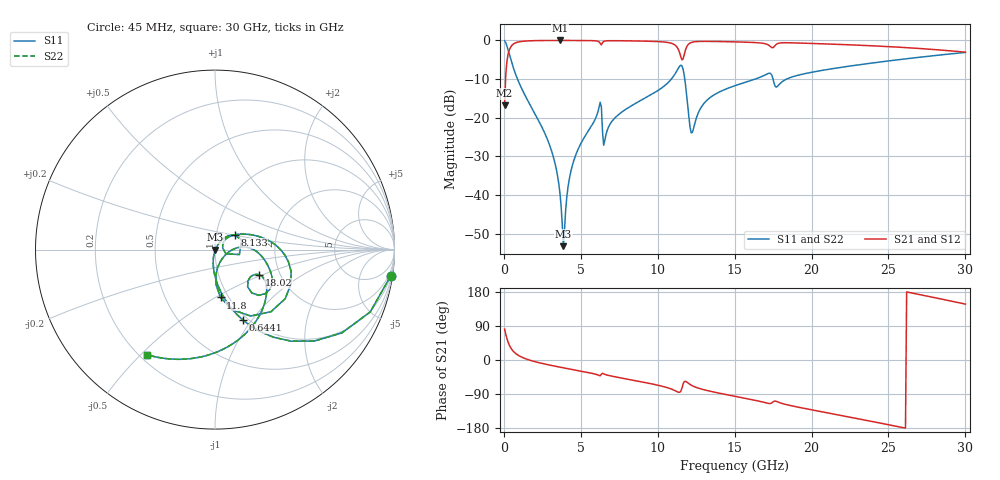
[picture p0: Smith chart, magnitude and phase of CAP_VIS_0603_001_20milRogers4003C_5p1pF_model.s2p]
! S-parameter model data by Modelithics Inc.  support@modelithics.com  813-866-6335  Tampa FL USA
! S-Parameter data specifications:
! Substrate: 20-mil Rogers 4003C, substrate thickness, H=0.508mm, Dielectric constant, Er=3.75
! PCB Mounting Pad Footprint: Pad width, PadW=0.90mm , Pad length, PadL=1.00mm , Pad gap, PadG (edge-to-edge)=1.00mm , Reference planes=3.0mm apart
! Created Wed Nov 18 13:23:11 2015
# hz S ma R 50
! 2 Port Network Data from SP1.SP block
! freq  magS11  angS11  magS21  angS21  magS12  angS12  magS22  angS22
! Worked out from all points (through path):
!   401 points, 45 MHz to 30 GHz, reference 50 ohm
!   highest |S21| = -0.02 dB at 3.64 GHz (marker M1); lowest = -16.8 dB at 45 MHz (marker M2)
!   group delay of S21, straight-line fit = 20.5 ps
!   lowest |S11| = -53.2 dB at 3.864 GHz (marker M3), VSWR 1.00, Z = 50.2 - j0.117 ohm
!   |S11| at or under -10 dB: 881.8 MHz to 10.89 GHz (10 GHz wide, 170 % of centre); 11.75 GHz to 16.34 GHz (4.588 GHz wide, 32.7 % of centre); 17.5 GHz to 18.38 GHz (886.1 MHz wide, 4.94 % of centre)
!   |S22| runs from -53.2 to -0.1 dB; largest |S21 - S12| = 0
!   S11 on the Smith chart (normalised r, x): 45 MHz: 1, -13; 644.1 MHz: 0.95, -0.91; 8.133 GHz: 1.23, +0.20; 11.8 GHz: 0.92, -0.53; 18.02 GHz: 1.57, -0.48; 30 GHz: 0.23, -0.52
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4.5e7  0.9896 -8.5  0.1439 81.5  0.1439 81.5  0.9896 -8.5
2.696625e8  0.7522 -42.6  0.6586 47.3  0.6586 47.3  0.7522 -42.6
6.441e8  0.4234 -68.3  0.9051 21.6  0.9051 21.6  0.4234 -68.3
2.965612e9  0.04448 -101.0  0.9969 -13.4  0.9969 -13.4  0.04448 -101.0
3.6396e9  0.01067 -97.8  0.9976 -18.9  0.9976 -18.9  0.01067 -97.8
3.864262e9  0.002177 -32.5  0.9975 -20.7  0.9975 -20.7  0.002177 -32.5
4.388475e9  0.02165 59.1  0.9971 -24.7  0.9971 -24.7  0.02165 59.1
5.062462e9  0.04879 56.9  0.9956 -29.9  0.9956 -29.9  0.04879 56.9
6.185775e9  0.1362 35.6  0.9584 -40.7  0.9584 -40.7  0.1362 35.6
6.560212e9  0.05105 32.5  0.9811 -37.9  0.9811 -37.9  0.05105 32.5
8.13285e9  0.1364 36.9  0.9858 -51.4  0.9858 -51.4  0.1364 36.9
1.007992e10  0.2291 20.5  0.9634 -67.2  0.9634 -67.2  0.2291 20.5
1.135301e10  0.441 -15.9  0.7538 -85.2  0.7538 -85.2  0.441 -15.9
1.180234e10  0.2686 -83.3  0.7524 -56.2  0.7524 -56.2  0.2686 -83.3
1.225166e10  0.06464 -28.3  0.9483 -68.0  0.9483 -68.0  0.06464 -28.3
1.315031e10  0.1646 5.1  0.9711 -80.0  0.9711 -80.0  0.1646 5.1
1.50225e10  0.2595 -7.5  0.9565 -95.8  0.9565 -95.8  0.2595 -7.5
1.719424e10  0.374 -33.1  0.8715 -114.5  0.8715 -114.5  0.374 -33.1
1.8018e10  0.2844 -29.7  0.9285 -113.9  0.9285 -113.9  0.2844 -29.7
2.003996e10  0.3879 -42.8  0.9122 -131.7  0.9122 -131.7  0.3879 -42.8
2.505742e10  0.544 -81.9  0.8292 -171.2  0.8292 -171.2  0.544 -81.9
3e10  0.6984 -123.1  0.7033 147.5  0.7033 147.5  0.6984 -123.1
